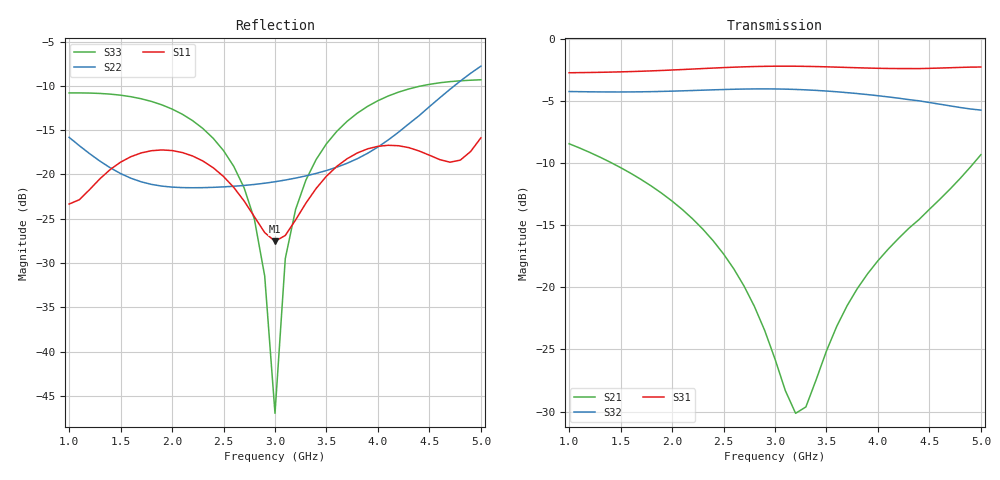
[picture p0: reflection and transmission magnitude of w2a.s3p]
# GHZ S RI R 50
!Output file by EM3DS 5.12 Built 2
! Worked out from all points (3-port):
!   41 points, 1 GHz to 5 GHz, reference 50 ohm
!   strongest paths, dB at 1 GHz, 2 GHz, 3 GHz, 4 GHz, 5 GHz:
!     S31: -2.7, -2.5, -2.2, -2.4, -2.3
!     S32: -4.2, -4.2, -4.0, -4.6, -5.7
!     S21: -8.4, -13.1, -25.8, -17.9, -9.3
!   lowest |S11| = -27.5 dB at 3 GHz (marker M1), VSWR 1.09, Z = 50.8 - j4.16 ohm
!   |S11| at or under -10 dB: start of sweep to end of sweep
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1  -0.0119 0.067  -0.1983 -0.3224  0.1517 -0.715
   -0.1983 -0.3224  0.1495 0.0623  0.0868 -0.608
   0.1517 -0.715  0.0868 -0.608  -0.2205 0.1861
1.7  -0.0291 0.129  -0.2701 0.0296  -0.4681 -0.5746
     -0.2701 0.0296  0.0905 -0.00872  -0.3973 -0.4662
     -0.4681 -0.5746  -0.3973 -0.4662  -0.1463 0.2238
2.2  0.0606 0.1117  -0.1146 0.1498  -0.7358 -0.1757
     -0.1146 0.1498  0.0688 -0.0484  -0.6026 -0.1458
     -0.7358 -0.1757  -0.6026 -0.1458  -0.0443 0.1962
2.6  0.0809 0.024  -0.00555 0.1186  -0.7349 0.2283
     -0.00555 0.1186  0.0224 -0.0828  -0.6025 0.1745
     -0.7349 0.2283  -0.6025 0.1745  0.0119 0.1103
2.9  0.0339 -0.0325  0.0181 0.0646  -0.5883 0.5057
     0.0181 0.0646  -0.0346 -0.0823  -0.4891 0.3961
     -0.5883 0.5057  -0.4891 0.3961  0.0078 0.0255
3  0.00963 -0.0408  0.0146 0.0493  -0.5143 0.582
   0.0146 0.0493  -0.0542 -0.073  -0.4315 0.4576
   -0.5143 0.582  -0.4315 0.4576  -0.00426 -0.00142
3.1  -0.0163 -0.0422  0.00691 0.0378  -0.43 0.647
     0.00691 0.0378  -0.0721 -0.0587  -0.3657 0.5105
     -0.43 0.647  -0.3657 0.5105  -0.0213 -0.0259
3.4  -0.0833 -0.00432  -0.0276 0.0323  -0.1357 0.762
     -0.0276 0.0323  -0.1008 0.0107  -0.1343 0.606
     -0.1357 0.762  -0.1343 0.606  -0.0952 -0.0755
4.3  0.0512 0.1321  0.0221 0.1715  0.6516 0.3908
     0.0221 0.1715  0.1716 0.0883  0.4685 0.3245
     0.6516 0.3908  0.4685 0.3245  -0.3034 0.0124
5  -0.00105 -0.1609  0.3064 0.1517  0.699 -0.3248
   0.3064 0.1517  0.1201 -0.3903  0.5053 -0.1098
   0.699 -0.3248  0.5053 -0.1098  -0.3157 0.1321
